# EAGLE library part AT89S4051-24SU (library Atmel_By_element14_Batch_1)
Microcontroller
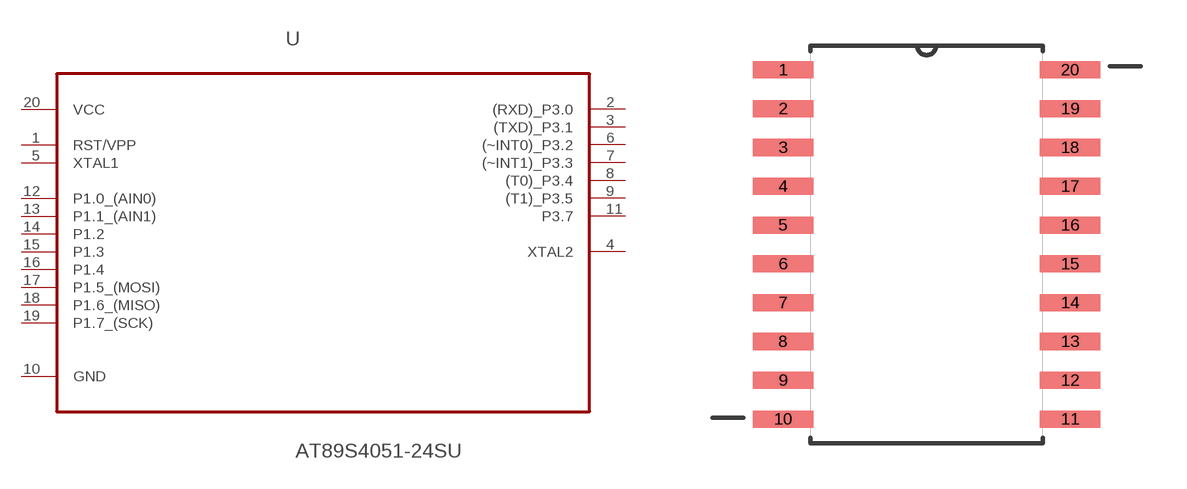
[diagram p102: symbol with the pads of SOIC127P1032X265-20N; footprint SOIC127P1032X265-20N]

Designator prefix U

## AT89S4051-24SU (DESCRIPTION: Microcontroller; MPN: AT89S4051-24SU; OC_FARNELL: 1095737; OC_NEWARK: 96K6576; PACKAGE: SOIC-20; SUPPLIER: ATMEL)  [SOIC127P1032X265-20N]
1  RST/VPP  pwr
2  (RXD)_P3.0
3  (TXD)_P3.1
4  XTAL2  out
5  XTAL1  in
6  (~INT0)_P3.2
7  (~INT1)_P3.3
8  (T0)_P3.4
9  (T1)_P3.5
10  GND  pas
11  P3.7
12  P1.0_(AIN0)
13  P1.1_(AIN1)
14  P1.2
15  P1.3
16  P1.4
17  P1.5_(MOSI)
18  P1.6_(MISO)
19  P1.7_(SCK)
20  VCC  pwr

## Footprint SOIC127P1032X265-20N (pad centres in mm)
smd 1.981 x 0.559: 1 -4.699,5.715; 2 -4.699,4.445; 3 -4.699,3.175; 4 -4.699,1.905; 5 -4.699,0.635; 6 -4.699,-0.635; 7 -4.699,-1.905; 8 -4.699,-3.175; 9 -4.699,-4.445; 10 -4.699,-5.715; 11 4.699,-5.715; 12 4.699,-4.445; 13 4.699,-3.175; 14 4.699,-1.905; 15 4.699,-0.635; 16 4.699,0.635; 17 4.699,1.905; 18 4.699,3.175; 19 4.699,4.445; 20 4.699,5.715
